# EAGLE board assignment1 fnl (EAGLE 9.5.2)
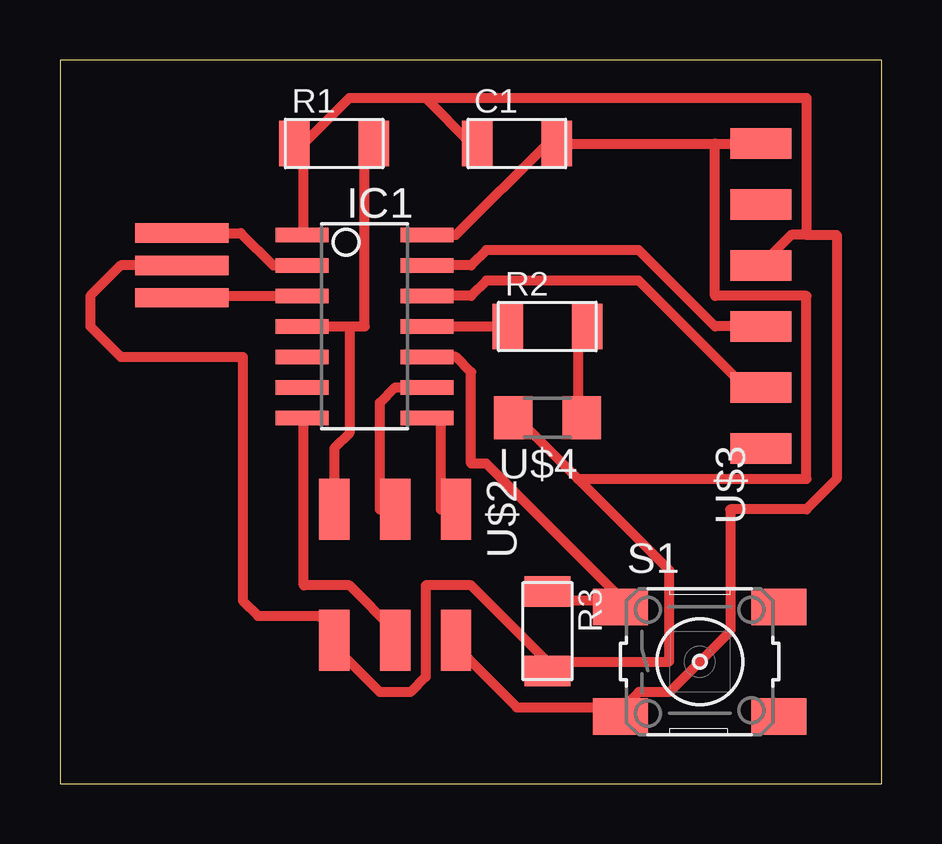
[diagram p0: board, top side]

Size 34.27 x 30.15 mm. Coordinates in mm from the lower left corner, seen from the top.
Outline: 0,0 34.27,0 34.27,30.15 0,30.15 0,0
Copper layers (1*16): Top 0.035mm / dielectric 1.5mm / Bottom 0.035mm
Design rules "default *": minimum track width 16mil, minimum drill 0.35mm, track to track 16mil, track to pad 16mil, pad to pad 16mil, via to via 16mil, smd to smd 16mil, copper to edge 40mil, drill to drill 16mil, minimum pad ring 10mil, minimum via ring 8mil, stop-mask expansion 4mil, vias tented up to drill 0mil, thermal gap 10mil

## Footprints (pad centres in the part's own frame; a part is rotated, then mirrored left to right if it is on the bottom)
C1206FAB = smd 1.27 x 1.905: 1 -1.651,0; 2 1.651,0
SOIC14 = smd 0.61 x 2.21: 1 -3.81,-2.603; 2 -2.54,-2.603; 3 -1.27,-2.603; 4 0,-2.603; 5 1.27,-2.603; 6 2.54,-2.603; 7 3.81,-2.603; 8 3.81,2.603; 9 2.54,2.603; 10 1.27,2.603; 11 0,2.603; 12 -1.27,2.603; 13 -2.54,2.603; 14 -3.81,2.603
R1206FAB = smd 1.27 x 1.905: 1 -1.651,0; 2 1.651,0
6MM_SWITCH = smd 2.286 x 1.524: 1 -3.302,2.286; 2 3.302,2.286; 3 -3.302,-2.286; 4 3.302,-2.286
EFOBM = smd 0.8 x 3.9: 1 -1.35,0; 2 0,0; 3 1.35,0
2X03SMD = smd 2.54 x 1.27: 1 -2.54,2.54; 2 2.92,2.54; 3 -2.54,0; 4 2.92,0; 5 -2.54,-2.54; 6 2.92,-2.54
1X06SMD = smd 2.54 x 1.27: 1 0,6.35; 2 0,3.81; 3 0,1.27; 4 0,-1.27; 5 0,-3.81; 6 0,-6.35
LED1206 = smd 1.6 x 1.803: 1 -1.422,0; 2 1.422,0

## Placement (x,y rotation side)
C1  [C1206FAB]  19.05,26.67 0 top
IC1  ATTINY44-SSU  [SOIC14]  12.7,19.05 270 top
R1  [R1206FAB]  11.43,26.67 0 top
R2  [R1206FAB]  20.32,19.05 0 top
R3  [R1206FAB]  20.32,6.35 270 top
S1  [6MM_SWITCH]  26.67,5.08 0 top
U$1  RESONATOR  [EFOBM]  5.08,21.59 270 top
U$2  CONN_03X2_AVRISPSMD  [2X03SMD]  13.97,8.89 270 top
U$3  CONN_06_FTDI-SMD-HEADER  [1X06SMD]  29.21,20.32 0 top
U$4  LED  [LED1206]  20.32,15.24 180 top

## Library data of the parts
C1 IC1 R1-R3 S1 U$1-U$4 = fab

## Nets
GND: C1.2 IC1.14 R3.2 U$1.2 U$2.6 U$3.1 U$4.2
LED: IC1.11 R2.1
MISO: IC1.8 U$2.1
MOSI: IC1.7 U$2.4
N$11: R2.2 U$4.1
RST: IC1.4 R1.2 U$2.5
RXD: IC1.12 U$3.5
SCK: IC1.9 U$2.3
SWITCH: IC1.10 R3.1 S1.1
TXD: IC1.13 U$3.4
VCC: C1.1 IC1.1 R1.1 S1.3 U$2.2 U$3.3
XTAL1: IC1.2 U$1.1
XTAL3: IC1.3 U$1.3

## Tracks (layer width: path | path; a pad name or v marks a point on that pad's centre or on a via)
GND
  Top 0.406: IC1.14 16.51,22.86 20.32,26.67 C1.2 27.3,26.67 | 27.3,26.67 U$3.1 | 21.59,12.7 25.4,8.89 25.4,5.08 20.32,5.08 | 21.59,12.7 19.05,15.24 U$4.2 | 20.32,5.08 17.14,8.26 15.24,8.26 15.24,4.45 14.61,3.81 13.33,3.81 11.43,5.71 U$2.6 11.43,6.35 10.79,6.99 8.26,6.99 7.62,7.62 7.62,17.78 2.54,17.78 1.27,19.05 1.27,20.32 2.54,21.59 U$1.2 | 20.32,5.08 R3.2 | 27.3,26.67 27.3,20.32 31.11,20.32 31.11,12.7 21.59,12.7
LED
  Top 0.406: IC1.11 R2.1
MISO
  Top 0.406: U$2.1 15.88,11.43 15.88,15.24 IC1.8
MOSI
  Top 0.406: IC1.7 10.16,15.24 10.16,8.26 12.06,8.26 13.97,6.35 U$2.4
N$11
  Top 0.406: U$4.1 21.59,15.24 21.59,19.05 R2.2
RST
  Top 0.406: IC1.4 12.06,19.05 | 12.06,19.05 12.7,19.05 12.7,26.67 R1.2 | U$2.5 11.43,13.97 12.06,14.61 12.06,19.05
RXD
  Top 0.406: IC1.12 17.14,20.32 17.78,20.96 24.13,20.96 28.57,16.51 U$3.5
SCK
  Top 0.406: IC1.9 13.97,16.51 13.33,15.88 13.33,11.43 U$2.3
SWITCH
  Top 0.406: R3.1 20.32,7.62 22.86,7.62 S1.1 23.5,7.62 17.78,13.34 17.14,13.34 17.14,17.14 16.51,17.78 IC1.10
TXD
  Top 0.406: IC1.13 17.14,21.59 17.78,22.23 24.13,22.23 27.3,19.05 U$3.4
VCC
  Top 0.406: U$2.2 16.51,5.71 19.05,3.18 22.86,3.18 S1.3 23.5,3.18 24.13,3.81 25.4,3.81 27.94,6.35 27.94,11.43 31.11,11.43 32.38,12.7 32.38,22.86 31.11,22.86 | 10.16,26.67 10.16,22.86 IC1.1 | 15.24,28.57 17.14,26.67 C1.1 | 15.24,28.57 12.06,28.57 10.16,26.67 | 10.16,26.67 R1.1 | U$3.3 30.48,22.86 31.11,22.86 | 31.11,22.86 31.11,28.57 15.24,28.57
XTAL1
  Top 0.406: IC1.2 8.89,21.59 7.54,22.94 U$1.1
XTAL3
  Top 0.406: U$1.3 5.16,20.32 IC1.3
